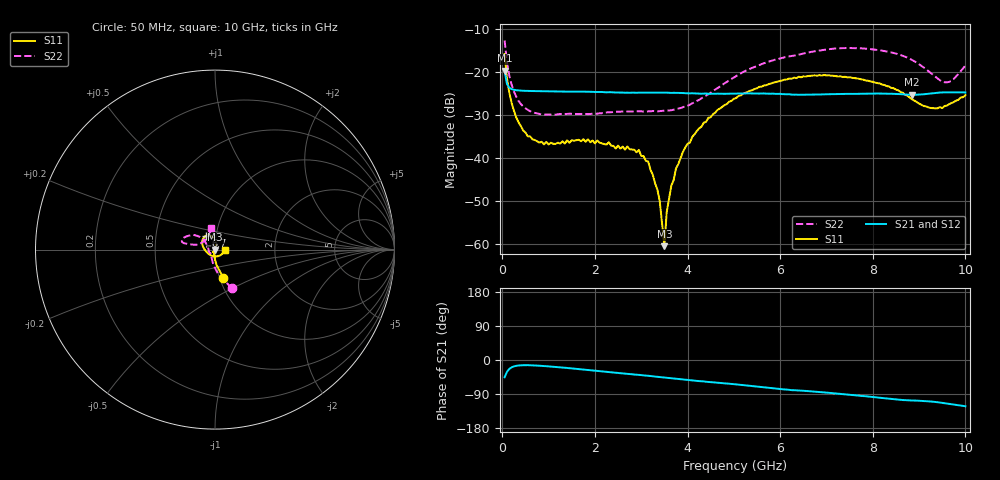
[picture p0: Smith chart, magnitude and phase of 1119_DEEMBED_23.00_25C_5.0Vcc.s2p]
!Hittite Microwave Corp.
!Digital Attenuator/PhaseShifter Rev 1.4.0
!Filename: C:\DATA\DATA\1119_DEEMBED_23.00_25C_5.0Vcc.s2p
!VNA ID: Agilent Technologies,N5224A,MY51441122,A.10.45.03
!Device type:
!2 Port Calibration.
!Temp(C): 25
!Lot Number:
!Serial Number:
!Operator:
!Misc:
!Attenuator:  23.000
# GHZ S DB R 50.0
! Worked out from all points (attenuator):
!   200 points, 50 MHz to 10 GHz, reference 50 ohm
!   highest |S21| = -19.63 dB at 50 MHz (marker M1); lowest = -25.2 dB at 8.85 GHz (marker M2)
!   lowest |S11| = -60.4 dB at 3.5 GHz (marker M3), VSWR 1.00, Z = 50.1 - j0.0496 ohm
!   |S11| at or under -10 dB: start of sweep to end of sweep
!   |S22| runs from -29.8 to -12.6 dB; largest |S21 - S12| = 0.0002
!   S11 on the Smith chart (normalised r, x): 50 MHz: 1.04, -0.33; 6.7 GHz: 0.90, +0.14; 10 GHz: 1.11, -0.01
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0.05  -15.79 -73.7  -19.63 -45.6  -19.63 -45.6  -12.60 -66.7
0.1  -21.34 -84.2  -22.70 -31.5  -22.70 -31.5  -17.55 -83.5
0.2  -27.07 -93.0  -23.89 -19.4  -23.90 -19.4  -22.83 -100.2
0.35  -31.60 -100.5  -24.21 -14.5  -24.22 -14.6  -26.62 -114.2
0.55  -34.86 -110.0  -24.32 -13.6  -24.32 -13.7  -28.71 -125.8
0.9  -36.75 -118.6  -24.39 -15.9  -24.39 -15.9  -29.81 -135.1
1.75  -35.53 -126.6  -24.50 -25.3  -24.50 -25.3  -29.67 -139.8
2.95  -38.05 -105.0  -24.72 -39.2  -24.73 -39.3  -29.08 -158.8
3.15  -40.71 -96.8  -24.73 -41.6  -24.74 -41.6  -29.07 -164.8
3.4  -49.90 -94.6  -24.72 -44.9  -24.73 -45.0  -29.01 -172.2
3.5  -60.39 -31.2  -24.71 -46.2  -24.71 -46.2  -28.91 -175.8
3.55  -52.50 52.6  -24.72 -47.2  -24.73 -47.2  -28.91 -177.6
3.65  -46.34 50.2  -24.79 -48.2  -24.79 -48.3  -28.81 178.7
3.9  -38.48 66.6  -24.81 -51.6  -24.82 -51.7  -28.11 168.1
4.45  -30.57 75.0  -24.99 -58.0  -25.00 -58.1  -25.09 147.4
5.05  -25.99 88.5  -24.95 -64.4  -24.96 -64.4  -20.86 139.4
6.7  -20.79 122.8  -25.15 -83.2  -25.16 -83.2  -15.20 154.5
8.35  -23.29 166.6  -24.99 -102.1  -24.99 -102.1  -15.25 168.2
8.85  -26.30 -164.8  -25.23 -106.9  -25.23 -106.8  -17.15 167.9
9.25  -28.29 -113.4  -24.93 -109.5  -24.94 -109.5  -20.14 162.4
9.55  -27.83 -65.1  -24.66 -114.1  -24.67 -114.2  -22.31 139.0
10  -25.29 -3.6  -24.69 -122.2  -24.69 -122.1  -18.41 99.6
